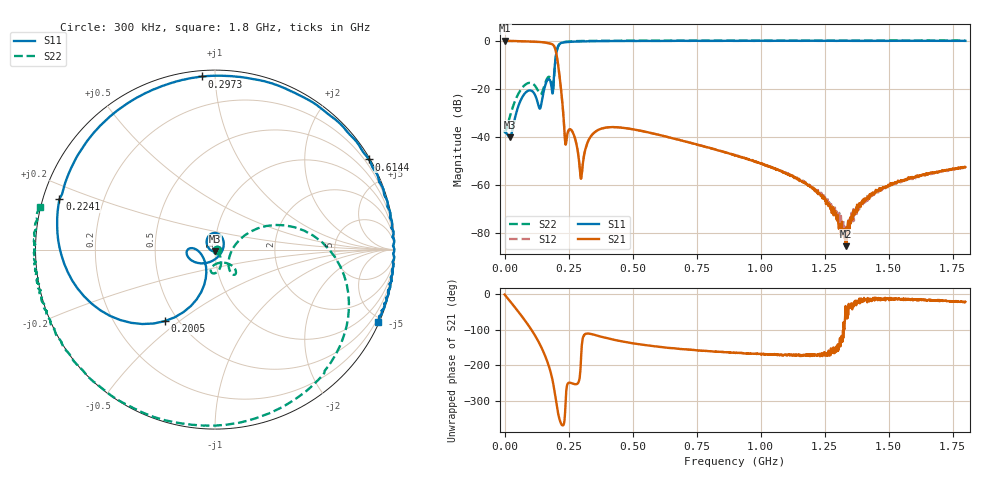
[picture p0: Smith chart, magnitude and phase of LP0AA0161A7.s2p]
!Agilent Technologies,E8358A,US40260310,A.06.04.32
!Agilent E8358A: A.06.04.32
!Date: Tuesday, October 15, 2019 06:07:02
!Correction: S11(Full 2 Port(1,2)) S21(Full 2 Port(1,2)) S12(Full 2 Port(1,2)) S22(Full 2 Port(1,2))
!S2P File: Measurements: S11, S21, S12, S22:
# Hz S  dB  R 50
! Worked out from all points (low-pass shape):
!   1601 points, 300 kHz to 1.8 GHz, reference 50 ohm
!   highest |S21| = -0.04 dB at 300 kHz (marker M1); lowest = -85.5 dB at 1.332 GHz (marker M2)
!   |S21| within 3 dB of the highest: start of sweep to 196.9 MHz
!   lowest |S11| = -40.1 dB at 20.55 MHz (marker M3), VSWR 1.02, Z = 50.2 - j0.971 ohm
!   |S11| at or under -10 dB: start of sweep to 196.6 MHz
!   |S22| runs from -38.6 to 0.1 dB; largest |S21 - S12| = 0.0087
!   S11 on the Smith chart (normalised r, x): 300 kHz: 1.03, +0.00; 200.5 MHz: 0.42, -0.44; 224.1 MHz: 0.05, +0.16; 297.3 MHz: 0.03, +0.93; 614.4 MHz: 0.05, +3.68; 1.8 GHz: 0.09, -4.71
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300000  -37.64 2.4  -0.04 -0.4  -0.11 -0.3  -38.62 1.1
2.054662e7  -40.13 -79.2  -0.07 -18.5  -0.14 -18.3  -31.69 -39.8
9.703388e7  -20.67 94.3  -0.33 -91.0  -0.38 -90.9  -17.54 -92.7
1.364023e8  -28.17 -21.3  -0.49 -138.3  -0.52 -138.2  -21.88 -87.1
1.543993e8  -20.43 -127.2  -0.68 -166.0  -0.72 -165.9  -19.08 -45.8
1.858941e8  -21.26 -169.7  -1.46 123.8  -1.49 123.8  -19.29 -46.2
2.005166e8  -6.23 -125.1  -4.41 62.3  -4.44 62.3  -6.73 15.7
2.241377e8  -0.81 162.0  -23.88 -8.3  -23.91 -8.3  -0.81 -48.0
2.387602e8  -0.59 139.5  -43.32 61.4  -43.33 61.4  -0.44 -64.8
2.680054e8  -0.40 111.9  -38.47 108.2  -38.51 108.1  -0.19 -86.6
2.972505e8  -0.29 94.3  -56.65 157.2  -57.09 158.9  -0.13 -100.2
3.006249e8  -0.28 92.6  -56.44 -155.2  -56.74 -153.8  -0.12 -101.4
3.276204e8  -0.25 81.3  -41.56 -110.4  -41.54 -110.0  -0.07 -110.3
3.714881e8  -0.18 67.6  -36.86 -117.9  -36.87 -117.8  -0.04 -121.0
6.009499e8  -0.08 31.8  -39.12 -147.4  -39.17 -147.5  -0.00 -148.5
6.144476e8  -0.06 30.4  -39.49 -148.5  -39.52 -148.2  -0.01 -149.3
9.0015e8  -0.07 10.5  -47.71 -164.4  -47.59 -163.9  0.05 -163.2
1.200475e9  -0.01 -2.9  -61.01 -169.7  -61.21 -171.5  0.01 -172.7
1.332078e9  -0.02 -7.9  -85.53 -32.7  -80.42 -76.8  0.02 -176.1
1.401816e9  -0.03 -10.4  -65.96 -19.8  -67.09 -17.9  0.03 -177.8
1.5008e9  -0.07 -13.5  -60.09 -12.0  -60.04 -15.2  0.09 179.2
1.8e9  -0.07 -23.9  -52.61 -20.7  -52.80 -23.0  0.02 166.4
